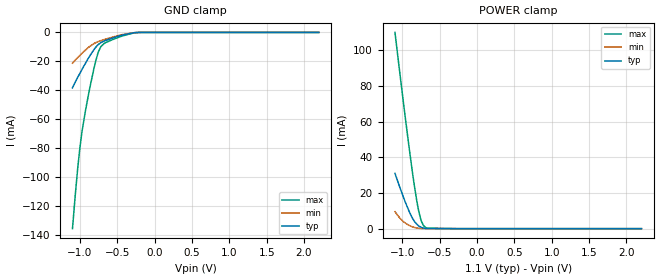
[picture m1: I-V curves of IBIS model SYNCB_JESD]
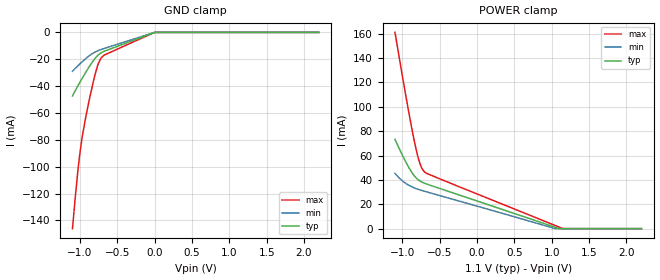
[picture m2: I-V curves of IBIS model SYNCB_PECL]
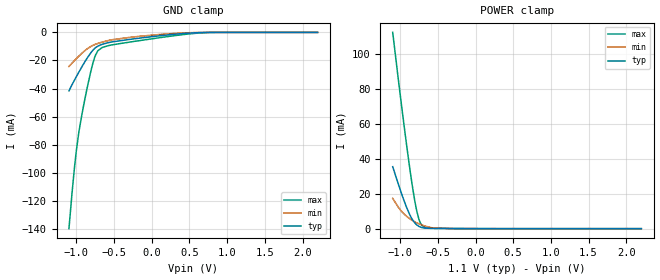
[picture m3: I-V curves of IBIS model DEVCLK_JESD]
| Texas Instruments Incorporated
| Up to 6.4-GSPS Single or 3.2-GSPS Dual Channel 12 bit ADC
| Marketing part#   Voltage Range   Package-type   #pins/pkg drawing
| ADC12DJ1600AAV   1.05V - 2.0V   BGA   144-pin AAV
| ADC12DJ2700AAV   1.05V - 2.0V   BGA   144-pin AAV
| ADC12DJ3200AAV   1.05V - 2.0V   BGA   144-pin AAV
[IBIS Ver]   4.1
[File name]   adc12djxx00.ibs
[File Rev]   1.1
[Date]   04/07/2017
[Source]   Model built from spectre simulations at:
   Texas Instruments Incorporated.
   Analog-eLab, HPA
   12500 TI Blvd
   Dallas, TX -75243
   For Support e-mail: elab_ibis@list.ti.com
[Notes]   Revision History
   Rev 1.1: 04/07/2017
   -Update package/pin RLC information
   Rev 1.0: 01/13/2015
   -Update OSCIN and CLKIN input buffer models
   -Pulldown non-monotonic for HSDS models
   -LVPECL simulation recommendation:
   It is recommended that a small (1nF or less) AC coupling cap
   be used. Larger values will result in long settling times
   - ccomp values are based on PVT settings:
   MIN: Low Voltage, High Temperature, Weak Process
   TYP: Nominal Voltage, Nominal Temperature, Nominal Process
   MAX: High Voltage, Low Temperature, Fast Process
   - C_comp although listed in numerical order of value are obtained from varying PVT conditions.
   For PVT conditions for each specific value, refer to the buffer description under respective [Model].
   IBIS model user is responsible for using appropriate C_comp to simulate for Signal Integrity.
[Disclaimer]  This model is designed as an aid for customers of Texas Instruments
 TI and its licensors and suppliers make no warranties, either expressed
 or implied, with respect to this  model, including the warranties of
 merchantability or fitness for a particular purpose.
 The model is provided solely on an "as is" basis. The entire risk as to
 its quality and performance is with the customer.
[Copyright] (C)Copyright 2017 Texas Instruments Incorporated.
   All rights reserved.
[Component]   ADC12DJxx00AAV
[Manufacturer]  Texas Instruments Incorporated
[Package]   |144-pin BGA AAV package
|   typ   min   max
R_pkg   0.5917   1.7313   0.9453
L_pkg   0.1861n   0.7116n   0.5998n
C_pkg   1.3757p   3.1822p   1.7136p
[Pin]   signal_name   model_name   R_pin   L_pin   C_pin
A1   AGND   GND
A2   AGND   GND
A3   AGND   GND
A4   INA+   NC   0.7444  2.154E-09   8.829E-13
A5   INA-   NC   0.7461  2.151E-09   8.780E-13
A6   AGND   GND
A7   AGND   GND
A8   DA3+   NC   0.6207  1.916E-09   8.569E-13
A9   DA3-   NC   0.7958  1.947E-09   9.025E-13
A10   DA2+   NC   0.8180  2.236E-09   1.022E-12
A11   DA2-   NC   0.9733  2.270E-09   1.076E-12
A12   DGND   GND
B1   TMSTP+   SYNCB   1.0765  2.813E-09   1.500E-12
B2   AGND   GND
B3   AGND   GND
B4   AGND   GND
B5   AGND   GND
B6   AGND   GND
B7   AGND   GND
B8   DA7+   NC   0.4513  1.386E-09   7.065E-13
B9   DA7-   NC   0.5020  1.503E-09   7.488E-13
B10   DA6+   NC   0.5131  1.557E-09   7.699E-13
B11   DA6-   NC   0.5736  1.671E-09   8.150E-13
B12   DGND   GND
C1   TMSTP-   SYNCB   0.9062  2.931E-09   1.469E-12
C2   SYNCSE\   INPUT   0.6609  1.978E-09   1.451E-12
C3   BG   NC   0.1861  7.116E-10   7.217E-13
C4   VA19   POWER
C5   VA11   POWER
C6   SCANEN   INPUT
C7   NCOA0   NC
C8   ORA0   NC
C9   VD11   POWER
C10   VD11   POWER
C11   DA5+   NC   0.5249  1.391E-09   7.391E-13
C12   DA1+   NC   0.6011  1.668E-09   8.346E-13
D1   AGND   GND
D2   VA11   POWER
D3   VA11   POWER
D4   VA19   POWER
D5   VA11   POWER
D6   AGND   GND
D7   NCOA1   NC
D8   ORA1   NC
D9   DGND   GND
D10   DGND   GND
D11   DA5-   NC   0.5079  1.559E-09   7.711E-13
D12   DA1-   NC   0.6053  1.872E-09   8.754E-13
E1   AGND   GND
E2   VA19   POWER
E3   VA19   POWER
E4   VA19   POWER
E5   VA11   POWER
E6   AGND   GND
E7   CALTRG   INPUT   0.2686  9.803E-10   9.049E-13
E8   SCS\   INPUT   0.3452  1.276E-09   1.154E-12
E9   VD11   POWER
E10   VD11   POWER
E11   DA4+   NC   0.3503  1.141E-09   6.077E-13
E12   DA0+   NC   0.4643  1.625E-09   7.716E-13
F1   CLK+   DEVCLK   1.3757  3.182E-09   1.709E-12
F2   AGND   GND
F3   AGND   GND
F4   VA19   POWER
F5   VA11   POWER
F6   AGND   GND
F7   CALSTAT   OUTPUT   0.3050  1.112E-09   1.061E-12
F8   SCLK   INPUT   0.2672  1.044E-09   9.163E-13
F9   DGND   GND
F10   DGND   GND
F11   DA4-   NC   0.3390  1.281E-09   6.306E-13
F12   DA0-   NC   0.5610  1.624E-09   7.916E-13
G1   CLK-   DEVCLK   1.1188  3.036E-09   1.714E-12
G2   AGND   GND
G3   AGND   GND
G4   VA19   POWER
G5   VA11   POWER
G6   AGND   GND
G7   VD11   POWER
G8   SDI   INPUT   0.2761  1.024E-09   1.068E-12
G9   DGND   GND
G10   DGND   GND
G11   DB4-   NC   0.3665  1.186E-09   6.237E-13
G12   DB0-   NC   0.5526  1.629E-09   7.855E-13
H1   AGND   GND
H2   VA19   POWER
H3   VA19   POWER
H4   VA19   POWER
H5   VA11   POWER
H6   AGND   GND
H7   VD11   POWER
H8   SDO   OUTPUT   0.2043  8.137E-10   8.609E-13
H9   VD11   POWER
H10   VD11   POWER
H11   DB4+   NC   0.3357  1.142E-09   5.998E-13
H12   DB0+   NC   0.4913  1.564E-09   7.605E-13
J1   AGND   GND
J2   VA11   POWER
J3   VA11   POWER
J4   VA19   POWER
J5   VA11   POWER
J6   AGND   GND
J7   NCOB1   NC
J8   ORB1   NC
J9   DGND   GND
J10   DGND   GND
J11   DB5-   NC   0.5188  1.535E-09   7.718E-13
J12   DB1-   NC   0.6166  1.836E-09   8.610E-13
K1   SYSREF+   SYSREF   0.9035  2.563E-09   1.554E-12
K2   TDIODE+   NC   0.4329  1.498E-09   1.181E-12
K3   TDIODE-   NC   0.4450  1.392E-09   1.153E-12
K4   VA19   POWER
K5   VA11   POWER
K6   PD   INPUT   0.4396  1.360E-09   9.496E-13
K7   NCOB0   NC
K8   ORB0   NC
K9   VD11   POWER
K10   VD11   POWER
K11   DB5+   NC   0.5500  1.481E-09   7.432E-13
K12   DB1+   NC   0.5734  1.718E-09   8.419E-13
L1   SYSREF-   SYSREF   0.9189  2.510E-09   1.518E-12
L2   AGND   GND
L3   AGND   GND
L4   AGND   GND
L5   AGND   GND
L6   AGND   GND
L7   AGND   GND
L8   DB7+   NC   0.4288  1.212E-09   6.660E-13
L9   DB70   NC   0.4697  1.411E-09   7.100E-13
L10   DB6+   NC   0.5079  1.550E-09   7.691E-13
L11   DB60   NC   0.5651  1.689E-09   8.183E-13
L12   DGND   GND
M1   AGND   GND
M2   AGND   GND
M3   AGND   GND
M4   INB+   NC   0.8858  2.154E-09   8.820E-13
M5   INB-   NC   0.7518  2.196E-09   8.857E-13
M6   AGND   GND
M7   AGND   GND
M8   DB3+   NC   0.6223  1.874E-09   8.453E-13
M9   DB3-   NC   0.7052  1.870E-09   8.988E-13
M10   DB2+   NC   0.7860  2.185E-09   1.012E-12
M11   DB2-   NC   0.8080  2.348E-09   1.063E-12
M12   DGND   GND
[Diff pin]  inv_pin  vdiff  tdelay_typ  tdelay_min  tdelay_max
A4   A5   0.0   0.0s   0.0s   0.0s
A8   A9   0.0   0.0s   0.0s   0.0s
A10   A11   0.0   0.0s   0.0s   0.0s
B8   B9   0.0   0.0s   0.0s   0.0s
B10   B11   0.0   0.0s   0.0s   0.0s
C1   B1   0.0   0.0s   0.0s   0.0s
D11   C11   0.0   0.0s   0.0s   0.0s
D12   C12   0.0   0.0s   0.0s   0.0s
F11   E11   0.0   0.0s   0.0s   0.0s
F12   E12   0.0   0.0s   0.0s   0.0s
G1   F1   0.0   0.0s   0.0s   0.0s
H11   G11   0.0   0.0s   0.0s   0.0s
H12   G12   0.0   0.0s   0.0s   0.0s
K11   J11   0.0   0.0s   0.0s   0.0s
K12   J12   0.0   0.0s   0.0s   0.0s
K1   L1   0.0   0.0s   0.0s   0.0s
L8   L9   0.0   0.0s   0.0s   0.0s
L10   L11   0.0   0.0s   0.0s   0.0s
M4   M5   0.0   0.0s   0.0s   0.0s
M8   M9   0.0   0.0s   0.0s   0.0s
M10   M11   0.0   0.0s   0.0s   0.0s
[Model Selector] SYNCB
SYNCB_JESD   Input configured for JESD204B LVDS levels
SYNCB_PECL   Input configured for LVCMOS levels
[Model Selector] DEVCLK
DEVCLK_JESD   Input configured for JESD204B LVDS levels
DEVCLK_PECL   Input configured for LVCMOS levels
[Model Selector] SYSREF
SYSREF_JESD   Input configured for JESD204B LVDS levels
SYSREF_PECL   Input configured for LVCMOS levels
| Models and submodels in the file (8): SYNCB_JESD (Input), SYNCB_PECL (Input), DEVCLK_JESD (Input), DEVCLK_PECL (Input), SYSREF_JESD (Input), SYSREF_PECL (Input), INPUT (Input), OUTPUT (3-state)
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|   Model SYNCB_JESD
[Model]   SYNCB_JESD
Model_type   Input
Vinl = .57
Vinh = 1.33
|   (nom PVT)   (fast PVT)   (slow PVT)
|   typ   min   max
C_comp   0.804p   0.760p   0.851p
[Voltage Range]   1.1   1.05   1.15
[Temperature Range]   27   125   -40
[Power Clamp Reference]   1.1   1.05   1.15
[GND Clamp Reference]   0   0   0
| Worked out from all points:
|   GND clamp passes 1 mA (typ) near -0.35 V on its own axis
|   POWER clamp passes 1 mA (typ) near -0.76 V on its own axis
[GND Clamp]
|   Voltage   I(typ)   I(min)   I(max)
-1.1V     -38.35mA   -21.26mA   -135.8mA
-1.031V   -31.21mA   -17.49mA   -94.47mA
-1.001V   -28.34mA   -15.93mA   -80.05mA
-968mV    -25.21mA   -14.25mA   -67.2mA
-928.4mV  -21.56mA   -12.32mA   -54.89mA
-862.4mV  -15.8mA    -9.467mA   -37.05mA
-786.5mV  -10.18mA   -7.057mA   -19.36mA
-720.5mV  -7.098mA   -5.706mA   -9.867mA
-674.3mV  -5.925mA   -4.944mA   -7.56mA
-436.7mV  -1.925mA   -1.597mA   -2.529mA
-222.2mV  -53.71uA   -55.81uA   -83.38uA
2.2V      0A         0A         0A
[POWER Clamp]
|   Voltage   I(typ)   I(min)   I(max)
-1.1V     30.96mA    9.496mA    110mA
-1.037V   23.42mA    6.048mA    88.02mA
-964.7mV  15.2mA     3.207mA    63.2mA
-911.9mV  9.817mA    1.854mA    45.83mA
-872.3mV  6.379mA    1.116mA    33.45mA
-836mV    3.901mA    624.7uA    22.9mA
-789.8mV  1.806mA    247.6uA    11.45mA
-753.5mV  844.2uA    105.5uA    5.111mA
-720.5mV  359.1uA    46.09uA    1.923mA
-684.2mV  119.2uA    18.69uA    528.2uA
-275mV    1.918uA    1.014uA    5.44uA
2.2V      0A         0A         0A
|   Model SYNCB_PECL
[Model]   SYNCB_PECL
Model_type   Input
Vinl = .57
Vinh = 1.33
|   (nom PVT)   (fast PVT)   (slow PVT)
|   typ   min   max
C_comp   0.804p   0.760p   0.851p
[Voltage Range]   1.1   1.05   1.15
[Temperature Range]   27   125   -40
[Power Clamp Reference]   1.1   1.05   1.15
[GND Clamp Reference]   0   0   0
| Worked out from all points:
|   GND clamp passes 1 mA (typ) near -0.05 V on its own axis
[GND Clamp]
|   Voltage   I(typ)   I(min)   I(max)
-1.1V     -47.36mA   -28.94mA   -146.1mA
-1.064V   -43.44mA   -26.91mA   -123.4mA
-1.027V   -39.78mA   -24.92mA   -102.9mA
-1.001V   -37.18mA   -23.5mA    -90.19mA
-968mV    -34mA      -21.78mA   -77.28mA
-888.8mV  -26.68mA   -17.97mA   -53.87mA
-803mV    -19.72mA   -14.77mA   -32.52mA
-753.5mV  -16.73mA   -13.51mA   -23.17mA
-723.8mV  -15.47mA   -12.89mA   -19.64mA
-697.4mV  -14.65mA   -12.38mA   -17.86mA
-1.1mV    -22.9uA    -19.5uA    -27.67uA
2.2V      0A         0A         0A
[POWER Clamp]
|   Voltage   I(typ)   I(min)   I(max)
-1.1V     73.25mA    45.31mA    161mA
-997.7mV  59.95mA    39.02mA    124.1mA
-925.1mV  51.31mA    35.98mA    98.86mA
-872.3mV  45.92mA    34.29mA    81.5mA
-836mV    42.96mA    33.31mA    70.44mA
-796.4mV  40.55mA    32.41mA    59.87mA
-753.5mV  38.72mA    31.56mA    51.44mA
-737mV    38.17mA    31.26mA    49.29mA
-697.4mV  37.1mA     30.55mA    46.24mA
1.048V    1.071mA    30.02uA    2.521mA
1.147V    0A         0A         66.58uA
2.2V      0A         0A         0A
|   Model DEVCLK_JESD
[Model]   DEVCLK_JESD
Model_type   Input
Vinl = .57
Vinh = 1.33
|   typ   min   max
|   (nom PVT)   (slow PVT)   (fast PVT)
C_comp   1.800p   1.766p   1.839p
[Voltage Range]   1.1   1.05   1.15
[Temperature Range]   27   125   -40
[Power Clamp Reference]   1.1   1.05   1.15
[GND Clamp Reference]   0   0   0
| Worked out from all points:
|   POWER clamp passes 1 mA (typ) near -0.74 V on its own axis
[GND Clamp]
|   Voltage   I(typ)   I(min)   I(max)
-1.1V     -41.71mA   -24.28mA   -139.9mA
-1.06V    -37.42mA   -22mA      -115.2mA
-1.024V   -33.74mA   -19.96mA   -94.96mA
-1.001V   -31.46mA   -18.69mA   -83.9mA
-964.7mV  -27.95mA   -16.75mA   -69.84mA
-885.5mV  -20.66mA   -12.9mA    -46.68mA
-809.6mV  -14.53mA   -10.03mA   -27.76mA
-760.1mV  -11.49mA   -8.745mA   -18.07mA
-717.2mV  -9.796mA   -7.896mA   -13.12mA
-532.4mV  -6.796mA   -5.272mA   -8.924mA
589.6mV   -251.9uA   -106.3uA   -620.9uA
2.2V      0A         0A         0A
[POWER Clamp]
|   Voltage   I(typ)   I(min)   I(max)
-1.1V     35.42mA    17.32mA    112.2mA
-958.1mV  17.01mA    8.781mA    61.95mA
-908.6mV  11.41mA    6.832mA    45.55mA
-849.2mV  5.951mA    4.947mA    27.24mA
-806.3mV  3.263mA    3.862mA    15.72mA
-779.9mV  2.129mA    3.295mA    9.913mA
-746.9mV  1.169mA    2.667mA    4.702mA
-713.9mV  620.4uA    2.107mA    1.925mA
-667.7mV  293.9uA    1.42mA     638.6uA
-568.7mV  118.7uA    400.3uA    265.1uA
-275mV    18.9uA     5.771uA    73.17uA
2.2V      0A         0A         0A
